FUNCTION_BLOCK Tolerance
VAR_INPUT
	ENABLE:BOOL;
	STEP_TYPE:STRING;
	STEP_TIME:INT;
	TOL_V:BOOL;
	TOL_P:BOOL;
	SV:INT;
	PV:REAL;
	WARNING_RANGE:INT;
	ALARM_RANGE:INT;
	DELAY_TIME:INT;
	STABLE_TIME:INT;
	RST:BOOL;
END_VAR
VAR_OUTPUT
	STU_WARNING:BOOL;
	
	STU_ALARM:BOOL;
	
	//STU_TIMEOUT:BOOL;
	STABLE_DONE:BOOL;
END_VAR
VAR
	SV_SUB_WARNING_RANGE:INT;
	SV_ADD_WARNING_RANGE:INT;
	SV_DIV_WARNING_RANGE:INT;
	SV_MUL_WARNING_RANGE:INT;
	
	SV_SUB_ALARM_RANGE:INT;
	SV_ADD_ALARM_RANGE:INT;
	SV_DIV_ALARM_RANGE:INT;
	SV_MUL_ALARM_RANGE:INT;
	
	STU_WARNING_V:BOOL;
	STU_WARNING_P:BOOL;
	
	STU_ALARM_V:BOOL;
	STU_ALARM_P:BOOL;
	
	TON_DELAY_TIME:TON;
	TON_DELAY_TIME_PT:INT;
	
	TON_ALARM_P		:TON;
	TON_ALARM_V		:TON;
	TON_WARNING_P	:TON;
	TON_WARNING_V	:TON;
	TON_STABLE		:TON;
	
	TON_STABLE_IN	:BOOL;
END_VAR

//初始化
IF NOT ENABLE OR RST
	THEN 
	
	STU_WARNING:=FALSE;
	
	STU_ALARM:=FALSE;
	
	STU_WARNING_P:=FALSE;
	STU_ALARM_P:=FALSE;
	
	STU_WARNING_V:=FALSE;
	STU_ALARM_V:=FALSE;
	STABLE_DONE:=FALSE;
	TON_STABLE_IN:=FALSE;
		
END_IF;
IF NOT TOL_P
	THEN 
	STU_WARNING_P:=FALSE;
	STU_ALARM_P:=FALSE;
END_IF;

IF NOT TOL_V
	THEN
	STU_WARNING_V:=FALSE;
	STU_ALARM_V:=FALSE;
END_IF;

IF NOT ENABLE AND (STEP_TYPE =	'Stable')
	THEN
	STABLE_DONE:=TRUE;
END_IF

//RANGE计算
	SV_SUB_WARNING_RANGE:=SV-WARNING_RANGE;
	SV_ADD_WARNING_RANGE:=SV+WARNING_RANGE;
	SV_DIV_WARNING_RANGE:=SV*(100-WARNING_RANGE)/100;
	SV_MUL_WARNING_RANGE:=SV*(100+WARNING_RANGE)/100;
	
	SV_SUB_ALARM_RANGE:=SV-ALARM_RANGE;
	SV_ADD_ALARM_RANGE:=SV+ALARM_RANGE;
	SV_DIV_ALARM_RANGE:=SV*(100-ALARM_RANGE)/100;
	SV_MUL_ALARM_RANGE:=SV*(100+ALARM_RANGE)/100;

//RANGE判断	
TON_WARNING_P(
			IN:= TOL_P AND (PV<=SV_DIV_WARNING_RANGE OR PV>=SV_MUL_WARNING_RANGE)AND NOT RST,
			PT:= T#200MS, 
			Q=> STU_WARNING_P, 
			ET=> );	
TON_WARNING_V(
			IN:= TOL_V AND (PV<=SV_SUB_WARNING_RANGE OR PV>=SV_ADD_WARNING_RANGE)AND NOT RST	, 
			PT:= T#200MS, 
			Q=> STU_WARNING_V, 
			ET=> );
TON_ALARM_P(
			IN:= TOL_P AND (PV<=SV_DIV_ALARM_RANGE OR PV>=SV_MUL_ALARM_RANGE)AND NOT RST, 
			PT:= T#200MS, 
			Q=> STU_ALARM_P, 
			ET=> );
TON_ALARM_V(
			IN:= TOL_V AND (PV<=SV_SUB_ALARM_RANGE OR PV>=SV_ADD_ALARM_RANGE)AND NOT RST, 
			PT:= T#200MS, 
			Q=> STU_ALARM_V, 
			ET=> );
			
IF ENABLE
	THEN	
	//TIME MODE
	IF STEP_TYPE =	'Time'
		THEN
		TON_DELAY_TIME_PT:=DELAY_TIME;
		STU_WARNING:=(STU_WARNING_V OR STU_WARNING_P) AND TON_DELAY_TIME.Q;
		IF (STU_ALARM_V OR STU_ALARM_P) AND TON_DELAY_TIME.Q
		THEN
		STU_ALARM:=TRUE;
		END_IF
	END_IF;	
	
	//Stable MODE
	IF STEP_TYPE =	'Stable'
		THEN
		IF TON_WARNING_P.IN OR TON_WARNING_V.IN
		THEN
		STABLE_DONE:=FALSE;
		TON_STABLE_IN:=FALSE;
		ELSE
		TON_STABLE_IN:=TRUE;			
		END_IF;	
		IF TON_STABLE.Q 
		THEN
		STABLE_DONE:=TRUE;	
		END_IF
	END_IF

END_IF;


//TON
	TON_DELAY_TIME(IN:= ENABLE AND NOT RST, PT:= INT_TO_TIME(TON_DELAY_TIME_PT)*1000, Q=> , ET=> );

	TON_STABLE(IN:=TON_STABLE_IN,	PT:= INT_TO_TIME(STABLE_TIME)*1000, Q=> , ET=> );

END_FUNCTION_BLOCK
